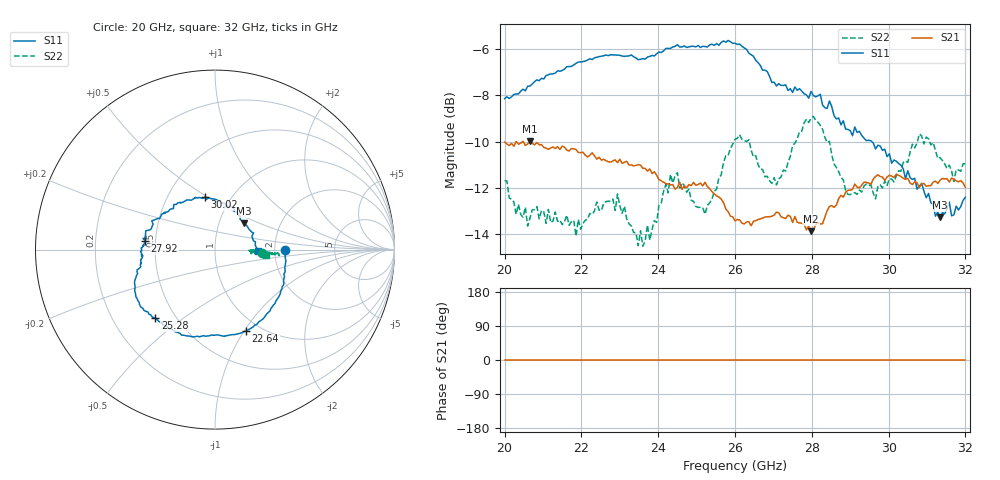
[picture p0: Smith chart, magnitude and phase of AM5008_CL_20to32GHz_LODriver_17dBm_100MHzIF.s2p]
!Keysight Technologies,N5245B,MY58422270,A.16.20.02
!Mixer S2P File: Scalar Mixer Measurement
!Calibration State: On
!Parameters: Stimulus Freq, S11, SC21, SC12, S22
# Hz  S  DB  R  50.0
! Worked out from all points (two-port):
!   201 points, 20 GHz to 32 GHz, reference 50 ohm
!   highest |S21| = -9.99 dB at 20.66 GHz (marker M1); lowest = -13.9 dB at 27.98 GHz (marker M2)
!   |S21| within 3 dB of the highest: start of sweep to 25.8 GHz; 28.4 GHz to end of sweep
!   lowest |S11| = -13.3 dB at 31.34 GHz (marker M3), VSWR 1.55, Z = 65.5 + j20.2 ohm
!   |S11| at or under -10 dB: 29.56 GHz to end of sweep
!   |S22| runs from -14.5 to -8.9 dB; largest |S21 - S12| = 0.32
!   S11 on the Smith chart (normalised r, x): 20 GHz: 2.29, -0.02; 22.64 GHz: 0.86, -1.02; 25.28 GHz: 0.39, -0.40; 27.92 GHz: 0.44, +0.05; 30.02 GHz: 0.76, +0.49; 32 GHz: 1.63, -0.03
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2e10  -8.15 -0.5  -10.02 0.0  -200.00 90.0  -11.69 -3.6
2.03e10  -7.94 -12.1  -9.99 0.0  -200.00 90.0  -13.14 -2.0
2.066e10  -7.60 -23.1  -9.99 0.0  -200.00 90.0  -13.30 -2.7
2.204e10  -6.55 -57.5  -10.46 0.0  -200.00 90.0  -13.54 -3.8
2.264e10  -6.27 -69.2  -10.82 0.0  -200.00 90.0  -12.59 -2.4
2.288e10  -6.26 -74.5  -10.79 0.0  -200.00 90.0  -12.97 -0.5
2.294e10  -6.26 -75.5  -10.90 0.0  -200.00 90.0  -12.26 -2.8
2.36e10  -6.42 -90.8  -11.15 0.0  -200.00 90.0  -14.51 -1.4
2.402e10  -6.14 -100.2  -11.64 0.0  -200.00 90.0  -12.74 -3.4
2.45e10  -5.82 -111.2  -11.98 0.0  -200.00 90.0  -11.34 -3.7
2.528e10  -5.92 -131.1  -11.94 0.0  -200.00 90.0  -12.75 -4.0
2.6e10  -5.76 -146.3  -13.42 0.0  -200.00 90.0  -9.90 -4.3
2.708e10  -7.60 -169.6  -13.04 0.0  -200.00 90.0  -11.87 -2.7
2.792e10  -8.13 172.8  -13.65 0.0  -200.00 90.0  -9.18 -2.8
2.798e10  -7.84 171.0  -13.87 0.0  -200.00 90.0  -8.99 -3.5
2.804e10  -8.01 171.3  -13.82 0.0  -200.00 90.0  -8.91 -5.3
2.894e10  -9.47 138.2  -12.10 0.0  -200.00 90.0  -12.27 -3.5
3.002e10  -10.52 100.6  -11.45 0.0  -200.00 90.0  -11.61 -3.3
3.08e10  -11.93 72.4  -11.99 0.0  -200.00 90.0  -9.67 -4.1
3.134e10  -13.27 42.5  -11.67 0.0  -200.00 90.0  -10.69 -3.8
3.17e10  -13.16 12.8  -11.61 0.0  -200.00 90.0  -11.72 -3.6
3.2e10  -12.40 -2.3  -11.97 0.0  -200.00 90.0  -10.96 -5.7
